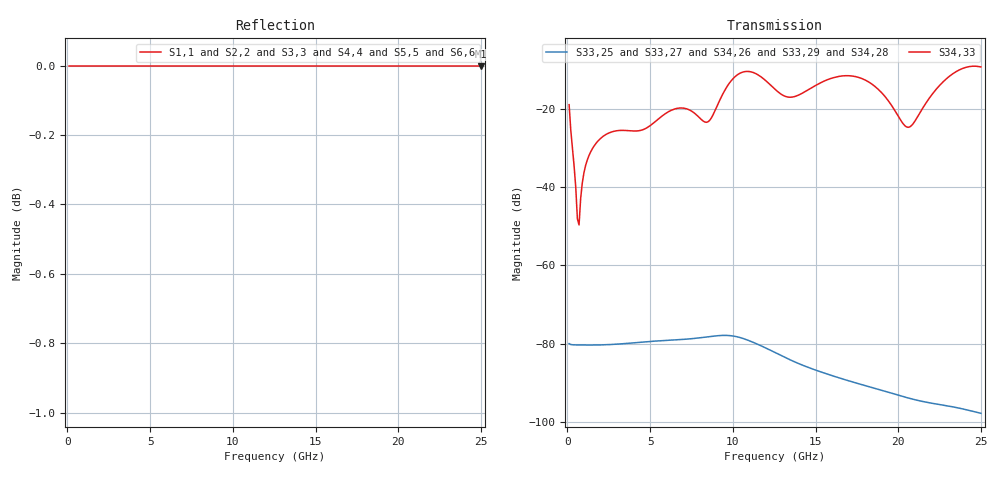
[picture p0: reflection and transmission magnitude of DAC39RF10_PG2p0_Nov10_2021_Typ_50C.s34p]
! Touchstone Ver. 1.0
! Number of ports is 34
# Hz	S	RI	R	50.000000
! SCATTERING PARAMETERS  :
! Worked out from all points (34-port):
!   250 points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, 100 MHz to 25 GHz, reference 50 ohm
!   strongest paths, dB at 100 MHz, 6.3 GHz, 12.6 GHz, 18.8 GHz, 25 GHz:
!     S34,33: -19.0, -20.3, -15.2, -15.1, -9.3
!     S33,25: -80.0, -79.1, -82.4, -91.6, -97.8
!     S33,27: -80.0, -79.1, -82.4, -91.7, -97.9
!     S34,26: -80.0, -79.1, -82.4, -91.6, -97.8
!     S33,29: -80.0, -79.1, -82.4, -91.7, -98.0
!     S34,28: -80.0, -79.1, -82.4, -91.7, -97.9
!   lowest |S11| = 0.0 dB at 25 GHz (marker M1)
!   |S11| at or under -10 dB: nowhere
